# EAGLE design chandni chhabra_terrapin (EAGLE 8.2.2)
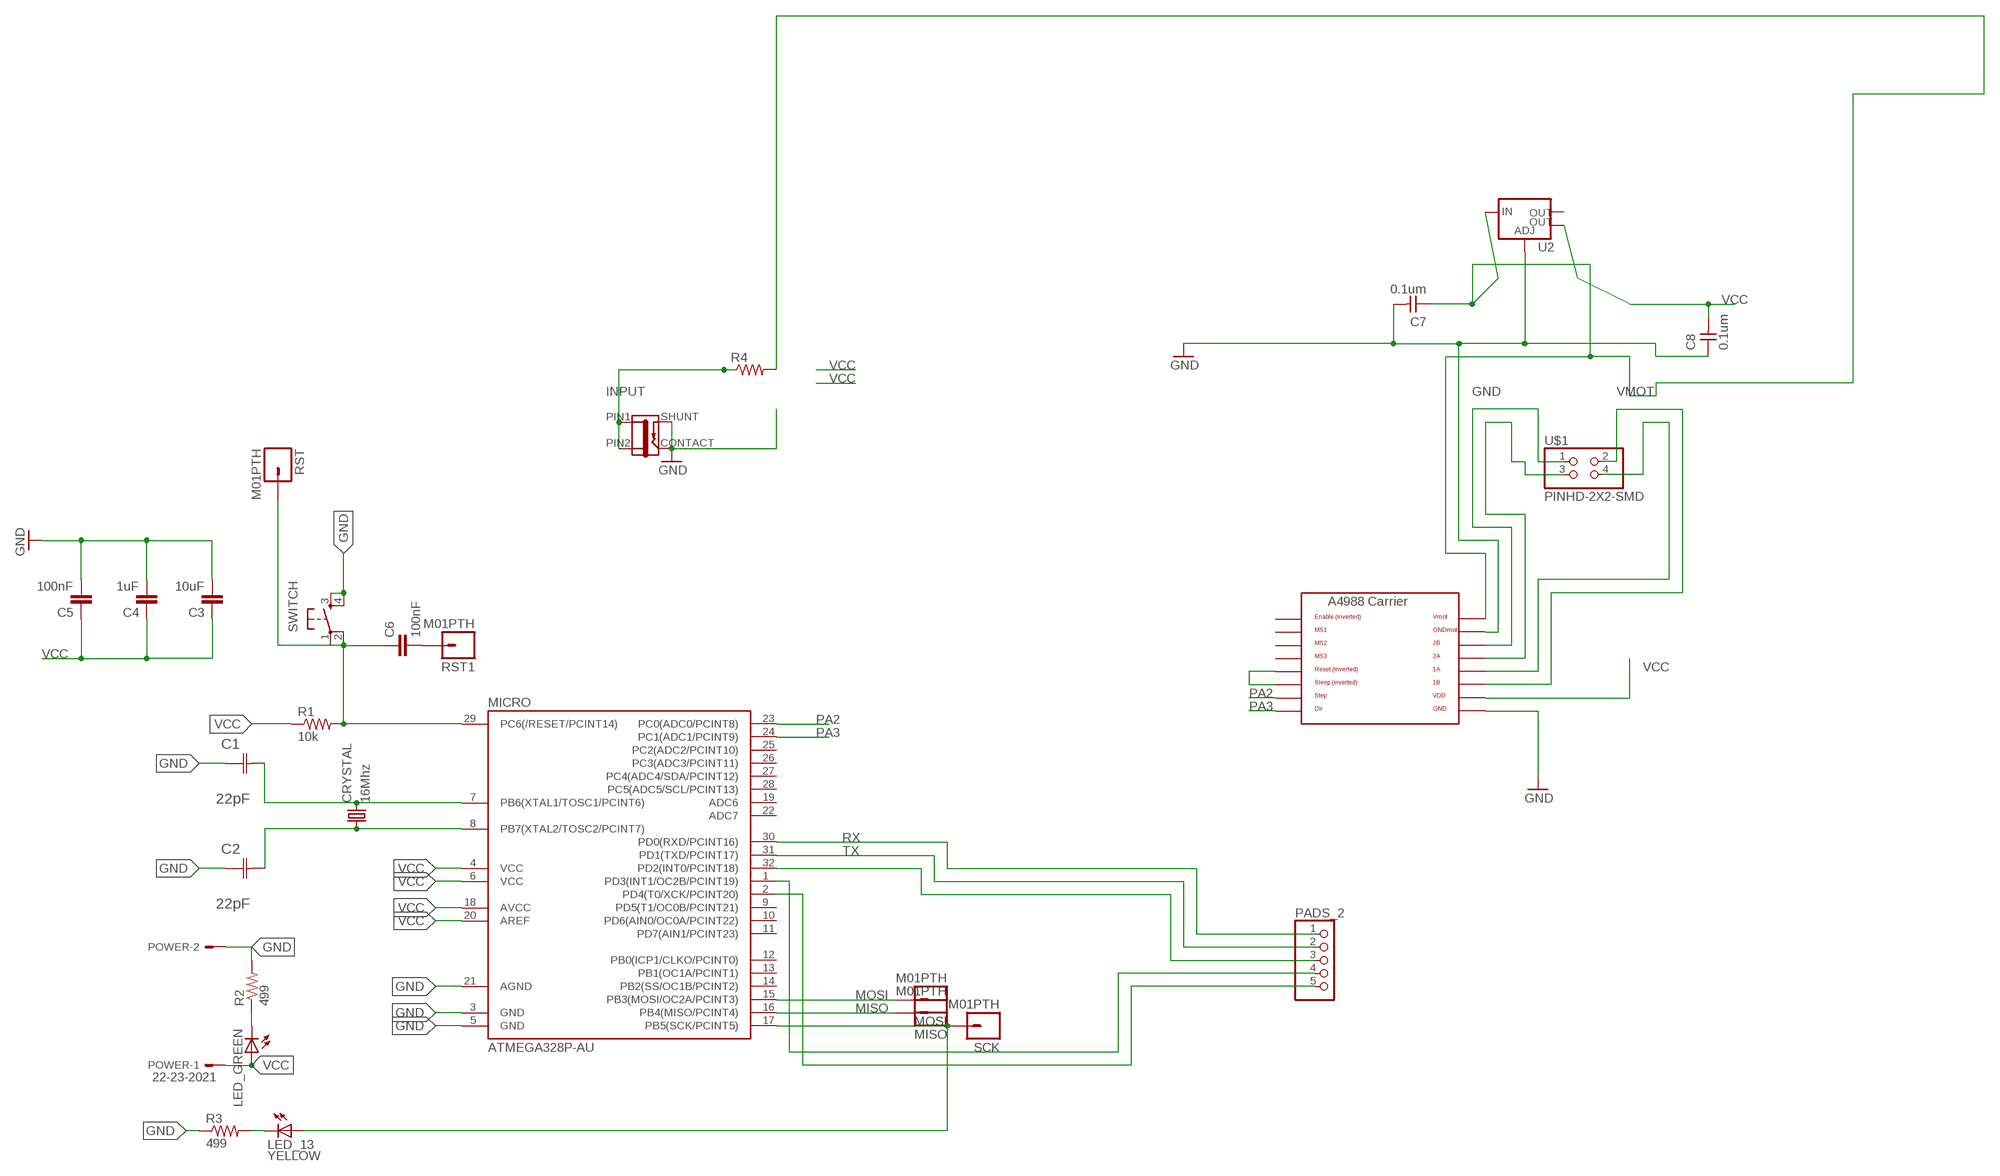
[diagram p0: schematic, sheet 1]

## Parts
C1  22pF  0612ZC225MAT2A  [CAPC3216X178N]
C2  22pF  0612ZC225MAT2A  [CAPC3216X178N]
C3  10uF  CAP1206  [1206]
C4  1uF  CAP1206  [1206]
C5  100nF  CAP1206  [1206]
C6  100nF  CAP1206  [1206]
C7  0.1um  CAP-UNPOLARIZEDFAB  [C1206FAB]
C8  0.1um  CAP-UNPOLARIZEDFAB  [C1206FAB]
CRYSTAL  16Mhz  CSM-7X-DU  [CSM-7X-DU]
J1  JACK-2.1MM  [PJ-002AH-SMT]
LED_13  YELLOW  LED1206  [1206]
LED_GREEN  LED1206  [1206]
MICRO  ATMEGA328P-AU  ATMEGA48/88/168-AU  [TQFP32-08]
MISO  M01PTH  [1X01]
MOSI  M01PTH  [1X01]
PADS_2  PINHD-1X5  [1X05]
POWER  22-23-2021  [22-23-2021]
R1  10k  RESISTOR1206  [1206]
R2  499  RESISTOR1206  [1206]
R3  499  RESISTOR1206  [1206]
R4  RES-US1206FAB  [R1206FAB]
RST  M01PTH  [1X01]
RST1  M01PTH  [1X01]
SCK  M01PTH  [1X01]
SWITCH  6MM_SWITCH6MM_SWITCH  [6MM_SWITCH]
U2  V_REG_LM1117SOT223  [SOT223]
U$1  PINHD-2X2-SMD  [2X02SMD]
U$2  A4988BREAKOUT  [A4988BREAKOUT]

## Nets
1A: U$1.4 U$2.1A
1B: U$1.2 U$2.1B
2A: U$1.3 U$2.2A
2B: U$1.1 U$2.2B
GND: C1.1(C1) C2.1(C1) C3.2 C4.2 C5.2 C7.2 C8.1 J1.CONTACT J1.SHUNT MICRO.3(GND) MICRO.5(GND) MICRO.21(AGND) POWER.2 R2.2 R3.1 SWITCH.3(S) SWITCH.4(S1) U2.1(ADJ) U$2.GND U$2.GNDMOT
INPUT: J1.PIN1 J1.PIN2 R4.1
MISO: MICRO.16(PB4(MISO/PCINT4)) MISO.1
MOSI: MICRO.15(PB3(MOSI/OC2A/PCINT3)) MOSI.1
N$2: C1.2(C2) CRYSTAL.2 MICRO.7(PB6(XTAL1/TOSC1/PCINT6))
N$9: C2.2(C2) CRYSTAL.1 MICRO.8(PB7(XTAL2/TOSC2/PCINT7))
N$13: C6.2 RST1.1
N$14: U$2.RST U$2.SLP(SLEEP)
N$22: MICRO.32(PD2(INT0/PCINT18)) PADS_2.3
N$23: MICRO.1(PD3(INT1/OC2B/PCINT19)) PADS_2.4
N$24: MICRO.2(PD4(T0/XCK/PCINT20)) PADS_2.5
N$26: LED_GREEN.2(C) R2.1
N$27: LED_13.2(C) R3.2
N$28: C6.1 MICRO.29(PC6(/RESET/PCINT14)) R1.2 RST.1 SWITCH.1(P) SWITCH.2(P1)
PA2: MICRO.23(PC0(ADC0/PCINT8)) U$2.STEP
PA3: MICRO.24(PC1(ADC1/PCINT9)) U$2.DIR
RX: MICRO.30(PD0(RXD/PCINT16)) PADS_2.1
SCK: LED_13.1(A) MICRO.17(PB5(SCK/PCINT5)) SCK.1
TX: MICRO.31(PD1(TXD/PCINT17)) PADS_2.2
VCC: C3.1 C4.1 C5.1 C8.2 LED_GREEN.1(A) MICRO.4(VCC) MICRO.6(VCC) MICRO.18(AVCC) MICRO.20(AREF) POWER.1 R1.1 U2.4(OUT) U$2.VDD
VMOT: C7.1 R4.2 U2.3(IN) U$2.VMOT
Unconnected: MICRO.9(PD5(T1/OC0B/PCINT21)) MICRO.10(PD6(AIN0/OC0A/PCINT22)) MICRO.11(PD7(AIN1/PCINT23)) MICRO.12(PB0(ICP1/CLKO/PCINT0)) MICRO.13(PB1(OC1A/PCINT1)) MICRO.14(PB2(SS/OC1B/PCINT2)) MICRO.19(ADC6) MICRO.22(ADC7) MICRO.25(PC2(ADC2/PCINT10)) MICRO.26(PC3(ADC3/PCINT11)) MICRO.27(PC4(ADC4/SDA/PCINT12)) MICRO.28(PC5(ADC5/SCL/PCINT13)) U2.2(OUT) U$2.EN U$2.MS1 U$2.MS2 U$2.MS3

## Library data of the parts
C1 C2 = AVX_By_element14_Batch_1:0612ZC225MAT2A: Capacitor 1206; MPN: 0612ZC225MAT2A; OC_FARNELL: -; OC_NEWARK: 12N3209; SUPPLIER: AVX; TOLERANCE: ±20%; VALUE: 2.2µF; VOLTAGERATING: 10V
C3-C6 = 01_SparkFun:CAP: Capacitor
C7 C8 = fab:CAP-UNPOLARIZED
CRYSTAL = 01_FAB_Hello:CSM-7X-DU: SMD CRYSTAL; OC_FARNELL: unknown; OC_NEWARK: unknown
J1 = fab:JACK-2.1MM: SMD DC power jack PJ-002AH-SMT As found in the fablab inventory. Made by Zaerc.
LED_13 LED_GREEN = 01_FAB_Hello:LED
MICRO = atmega8:ATMEGA48/88/168
MISO MOSI RST RST1 SCK = 01_SparkFun:M01: Header 1
PADS_2 = pinhead:PINHD-1X5: PIN HEADER
POWER = con-molex:22-23-2021: .100" (2.54mm) Center Header - 2 Pin; MF: MOLEX; MPN: 22-23-2021; OC_FARNELL: 1462926; OC_NEWARK: 25C3832
R1-R3 = 01_SparkFun:RESISTOR: Resistor
R4 = fab:RES-US: Resistor (US Symbol)
SWITCH = 01_FAB_Hello:6MM_SWITCH: OMRON SWITCH
U2 = fab:V_REG_LM1117: Voltage Regulator LM1117 Standard adjustable voltage regulator but in SMD form. Spark Fun Electronics SKU : COM-00595; PROD_ID: VREG-08170
U$1 = fab:PINHD-2X2-SMD
U$2 = RepRapjr:A4988BREAKOUT

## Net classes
0 default: width 0.035 mm, clearance 0.4 mm

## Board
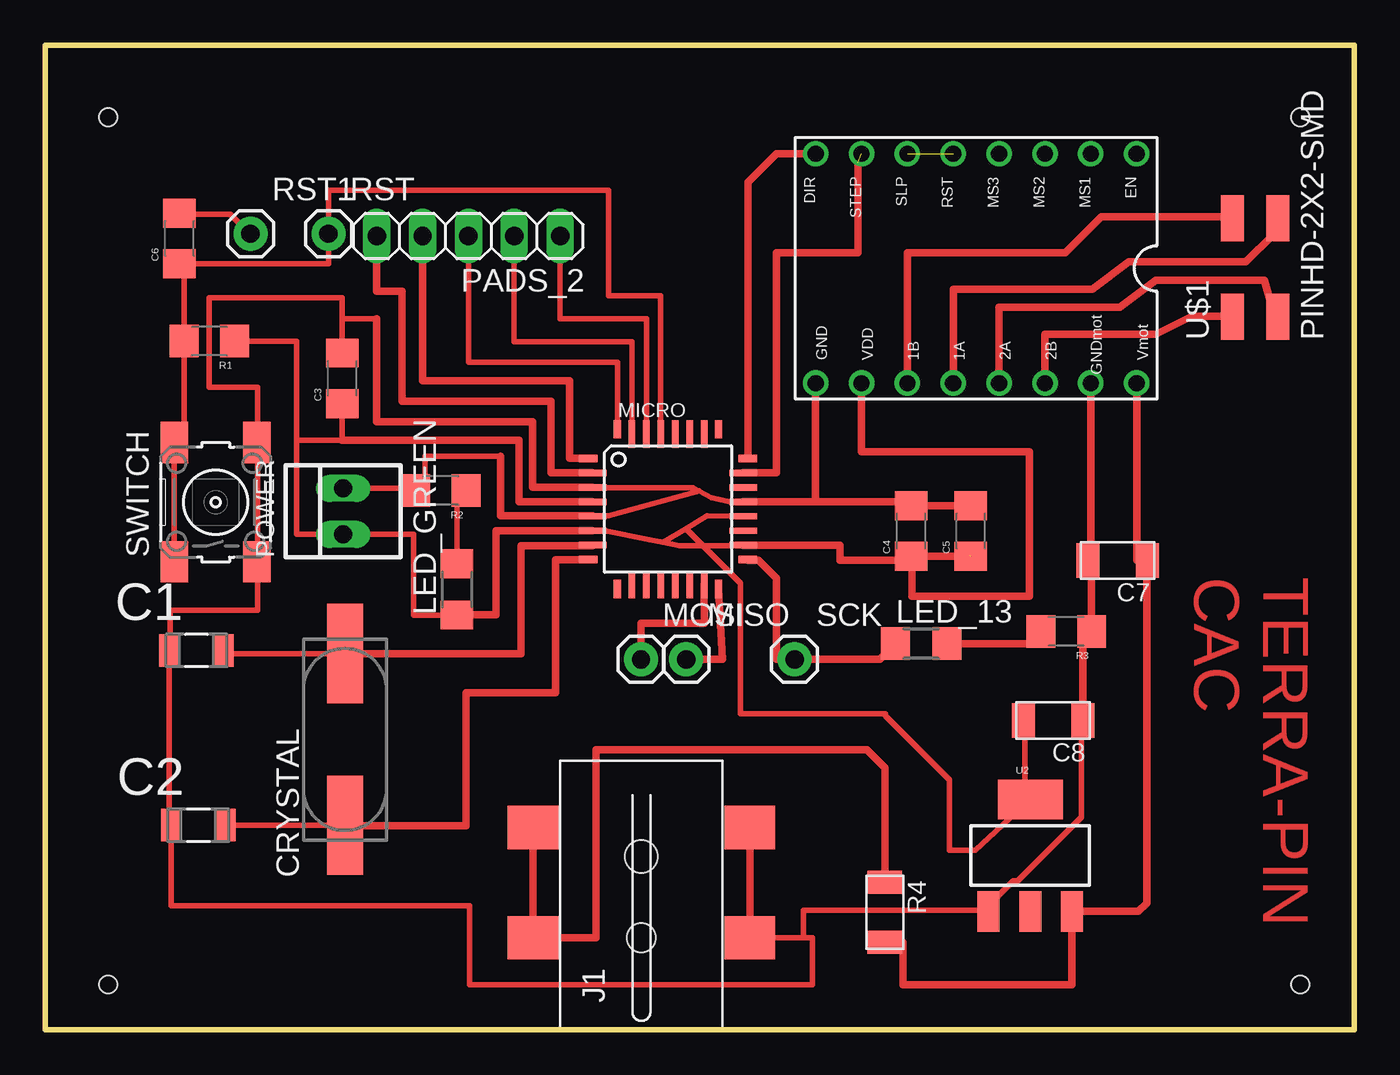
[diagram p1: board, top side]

Size 72.5 x 54.5 mm. Coordinates in mm from the lower left corner, seen from the top.
Outline: 72.5,54.5 0,54.5 0,0 72.5,0 72.5,54.5
Copper layers (1*16): Top 0.035mm / dielectric 1.5mm / Bottom 0.035mm
Design rules "fab": minimum track width 0.3mm, minimum drill 32mil, track to track 0.315mm, track to pad 0.315mm, pad to pad 0.315mm, via to via 0.315mm, smd to smd 0.315mm, copper to edge 40mil, drill to drill 16mil, minimum pad ring 10mil, minimum via ring 8mil, stop-mask expansion 4mil, vias tented up to drill 0mil, thermal gap 10mil
Holes 1 mm at 3.5,50.5 3.5,2.5 69.5,2.5 69.5,50.5

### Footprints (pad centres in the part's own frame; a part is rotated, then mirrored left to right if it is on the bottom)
CAPC3216X178N = smd 1.118 x 1.803: 1 -1.499,0; 2 1.499,0
1206 = smd 1.6 x 1.8: 1 -1.4,0; 2 1.4,0
C1206FAB = smd 1.27 x 1.905: 1 -1.651,0; 2 1.651,0
CSM-7X-DU = smd 5.5 x 2: 1 -4.75,0; 2 4.75,0
PJ-002AH-SMT = smd 2.4 x 2.8: CONTACT -2.4,-6; PIN1 3.7,6; PIN2 -2.4,6; SHUNT 3.7,-6 | hole 1.6: -2.4,0 | hole 1.8: 2.1,0
1206' = smd 1.6 x 1.803: 1 -1.422,0; 2 1.422,0
TQFP32-08 = smd 1.016 x 0.406: 1 -4.42,2.8; 8 -4.42,-2.8; 17 4.42,-2.8; 24 4.42,2.8 | smd 1.524 x 0.356: 2 -4.166,2; 3 -4.166,1.2; 4 -4.166,0.4; 5 -4.166,-0.4; 6 -4.166,-1.2; 7 -4.166,-2; 18 4.166,-2; 19 4.166,-1.2; 20 4.166,-0.4; 21 4.166,0.4; 22 4.166,1.2; 23 4.166,2 | smd 0.406 x 1.016: 9 -2.8,-4.42; 16 2.8,-4.42; 25 2.8,4.42; 32 -2.8,4.42 | smd 0.356 x 1.524: 10 -2,-4.166; 11 -1.2,-4.166; 12 -0.4,-4.166; 13 0.4,-4.166; 14 1.2,-4.166; 15 2,-4.166; 26 2,4.166; 27 1.2,4.166; 28 0.4,4.166; 29 -0.4,4.166; 30 -1.2,4.166; 31 -2,4.166
1X01 = drill 1.016 pad 1.88: 1 0,0
1X05 = drill 1.016 long: 1 -5.08,0; 2 -2.54,0; 3 0,0; 4 2.54,0; 5 5.08,0
22-23-2021 = drill 1 long: 1 -1.27,0; 2 1.27,0
R1206FAB = smd 1.27 x 1.905: 1 -1.651,0; 2 1.651,0
6MM_SWITCH = smd 2.286 x 1.524: 1 -3.302,2.286; 2 3.302,2.286; 3 -3.302,-2.286; 4 3.302,-2.286
SOT223 = smd 1.219 x 2.235: 1 -2.311,-3.099; 2 0,-3.099; 3 2.311,-3.099 | smd 3.6 x 2.2: 4 0,3.099
2X02SMD = smd 2.54 x 1.27: 1 -2.54,1.27; 2 2.92,1.27; 3 -2.54,-1.27; 4 2.92,-1.27
A4988BREAKOUT = drill 0.9: 1A 8.89,1.27; 1B 11.43,1.27; 2A 6.35,1.27; 2B 3.81,1.27; DIR 16.51,-11.43; EN -1.27,-11.43; GND 16.51,1.27; GNDMOT 1.27,1.27; MS1 1.27,-11.43; MS2 3.81,-11.43; MS3 6.35,-11.43; RST 8.89,-11.43; SLP 11.43,-11.43; STEP 13.97,-11.43; VDD 13.97,1.27; VMOT -1.27,1.27

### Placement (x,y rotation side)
C1  8.38,21 0 top
C2  8.48,11.32 0 top
C3  16.46,36.06 90 top
C4  47.95,27.61 90 top
C5  51.25,27.61 90 top
C6  7.44,43.81 90 top
C7  59.4,25.98 180 top
C8  55.83,17.12 180 top
CRYSTAL  16.61,16.07 90 top
J1  33.02,7.49 90 top
LED_13  YELLOW  [1206']  48.52,21.37 0 top
LED_GREEN  [1206']  22.81,24.38 90 top
MICRO  34.49,28.82 0 top
MISO  35.5,20.5 0 top
MOSI  33,20.5 0 top
PADS_2  23.44,43.93 180 top
POWER  16.51,28.69 90 top
R1  9.09,38.12 180 top
R2  21.92,29.84 180 top
R3  56.55,22.05 180 top
R4  46.5,6.5 270 top
RST  15.69,44.06 0 top
RST1  11.38,44.06 0 top
SCK  41.5,20.5 0 top
SWITCH  9.45,29.2 90 top
U2  54.56,9.64 0 top
U$1  67,42 90 top
U$2  59.18,37.06 180 top

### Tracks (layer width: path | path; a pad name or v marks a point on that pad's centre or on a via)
1A
  Top 0.406: U$2.1A 50.29,41 58,41 60,42.5 66.5,42.5 68,44 68,44.65 U$1.4
1B
  Top 0.406: U$2.1B 47.75,43 56.5,43 58.5,45 65.65,45 U$1.2
2A
  Top 0.406: U$2.2A 52.83,40 59.5,40 61.5,41.5 67.5,41.5 68,39.73 U$1.3
2B
  Top 0.406: U$2.2B 55.37,38.5 61.5,38.5 63.5,39.5 65.69,39.5 U$1.1
GND
  Top 0.305: MICRO.5 | MICRO.21 38.05,29.2 36.9,29.45 35.88,29.99 | C1.1 6.88,11.32 C2.1 6.98,6.85 23.5,6.85 23.5,2.5 42.5,2.5 42.5,5.09 42,5.09 | C1.1 6.8,21 | 25.22,31.74 21.03,31.74 21.03,29.71 21.02,29.71 R2.2 21.02,29.96 POWER.2 | 30.32,28.44 MICRO.5 | C1.1 6.93,21 6.93,23.23 11.76,23.23 11.76,25.9 | MICRO.5 30.93,28.44 31.19,28.44 36.06,29.79 | 18.36,39.36 16.46,39.36 | MICRO.3 30.35,29.99 35.88,29.99 | 36.06,29.79 36.2,29.82 | 35.88,29.99 36.06,29.79 | C3.2 16.46,39.36 | SWITCH.3 11.76,25.9 | 11.76,25.9 11.76,31.87 11.73,31.87 SWITCH.4 11.76,32.5 11.76,35.55 9.09,35.55 9.09,40.5 16.46,40.5 16.46,39.36 | 57.38,16.12 C8.1 57.38,16 57.38,11.75 53.88,8.25 53.62,8.25 52.12,6.75 U2.1 52.12,6.62 42,6.62 42,5.09 | 42,5.09 J1.CONTACT
  Top 0.406: 25.22,31.74 25.22,28.44 30.32,28.44 | MICRO.3 27,30.02 27,33.65 18.36,33.65 18.36,39.36 | J1.CONTACT J1.SHUNT | C8.1 57.48,21.58 R3.1 57.95,25.78 C7.2 57.91,25.98 U$2.GNDMOT | MICRO.21 42.5,29.22 42.67,29.22 | 42.67,29.22 U$2.GND | 42.67,29.22 47.95,29.22 C4.2 C5.2
INPUT
  Top 0.305: 27.5,5.09 J1.PIN2
  Top 0.406: 27.5,5.09 J1.PIN2 | J1.PIN2 J1.PIN1 | J1.PIN2 30.5,5.09 30.5,15.5 45.5,15.5 46.5,14.5 R4.1
MISO
  Top 0.406: MICRO.16 37.5,20.5 MISO.1
MOSI
  Top 0.406: MICRO.15 36.5,22.5 33,22.5 MOSI.1
N$2
  Top 0.305: 9.88,20.82 C1.2 9.88,20.82 | 30.32,26.79 MICRO.7 | CRYSTAL.2 9.88,20.82
  Top 0.406: 30.32,26.79 26.36,26.79 26.36,20.82 CRYSTAL.2
N$9
  Top 0.305: 9.98,11.29 C2.2 | MICRO.8 | C2.2 CRYSTAL.1 16.61,11.29 | C2.2
  Top 0.406: MICRO.8 28.27,26.03 28.27,18.66 23.31,18.66 23.31,11.29 16.61,11.29
N$13
  Top 0.305: C6.2 7.77,45.13 10.26,45.13 11.32,44.06 RST1.1
N$14  (1 unrouted)
N$22
  Top 0.305: MICRO.32 31.7,36.95 23.44,36.95 PADS_2.3
N$23
  Top 0.406: MICRO.1 29.03,31.62 29.03,35.93 20.9,35.93 PADS_2.4
N$24
  Top 0.406: MICRO.2 28.01,30.82 28.01,34.79 19.76,34.79 19.76,40.88 18.36,40.88 PADS_2.5
N$26
  Top 0.305: 23.7,29.58 R2.1 23.32,29.45 22.81,29.45 LED_GREEN.2
N$27
  Top 0.406: LED_13.2 54.47,21.37 R3.2
N$28
  Top 0.305: 34.11,32.99 MICRO.29 34.09,40.63 31.19,40.63 31.19,46.47 15.69,46.47 RST.1 15.69,42.41 7.69,42.41 | R1.2 7.44,38.12 | R1.2 7.69,32.5 SWITCH.2 SWITCH.1 | C6.1 7.69,42.41 | 7.69,42.41 R1.2
PA2  (1 unrouted)
  Top 0.406: MICRO.23 40.5,30.82 40.5,43 45,43 45,48
PA3
  Top 0.305: 39.06,31.61 MICRO.24
  Top 0.406: MICRO.24 38.91,46.91 40.5,48.5 42.66,48.5 U$2.DIR
RX
  Top 0.305: PADS_2.1 28.52,39.36 33.29,39.36 MICRO.30
SCK
  Top 0.406: LED_13.1 46.23,20.5 SCK.1 40.5,20.5 40.5,25 39.5,26 38.93,26 MICRO.17
TX
  Top 0.305: PADS_2.2 25.98,38.09 32.49,38.09 MICRO.31
VCC  (1 unrouted)
  Top 0.305: MICRO.18 38.66,26.79 35.12,26.79 34.22,26.97 | MICRO.20 36.65,28.44 35.49,27.74 | 13.92,32.63 13.92,38.12 R1.1 | 13.92,32.63 13.92,27.42 POWER.1 20.39,27.42 20.39,22.95 LED_GREEN.1 22.81,22.98 | MICRO.6 31.01,27.63 33.47,27.13 34.22,26.97 | 35.49,27.74 34.22,26.97 | 13.92,32.63 16.46,32.63 C3.1 16.84,34.66 16.84,34.41 | 35.49,27.74 35.51,27.7 38.5,24.71 38.5,17.5 46.53,17.5 46.53,17.39 50.09,13.83 50.09,9.92 51.51,9.92 U2.4 54.25,12.62 54.25,16 C8.2 | 51.25,26.5 51.25,26.25 | C5.1 51.51,26.28
  Top 0.406: MICRO.4 26.23,29.22 26.23,32.63 16.46,32.63 | MICRO.6 24.97,27.62 24.97,22.98 22.81,22.98 | MICRO.18 44,26.82 44,26 47.95,26 C4.1 | C4.1 48,26.21 48,24 54.5,24 54.5,32 45.21,32 U$2.VDD | C4.1 C5.1
VMOT
  Top 0.305: 56.88,6.62 U2.3
  Top 0.406: R4.2 47.5,4.85 47.5,2.5 56.87,2.5 U2.3 60.54,6.54 61,7 61,25.93 C7.1 60.45,25.98 U$2.VMOT

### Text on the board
Top: TERRA-PIN / CAC

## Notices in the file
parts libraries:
01_SparkFun: Licensing: CC v3.0 Share-Alike You are welcome to use this library for commercial purposes.
